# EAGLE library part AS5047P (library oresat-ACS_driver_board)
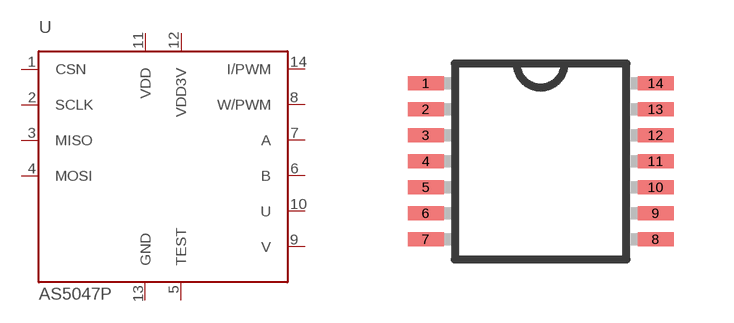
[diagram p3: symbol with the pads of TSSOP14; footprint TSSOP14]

Designator prefix U

## AS5047P  [TSSOP14]
1  CSN  in
2  SCLK  in
3  MISO  out
4  MOSI  in
5  TEST  pwr
6  B  out
7  A  out
8  W/PWM  out
9  V  out
10  U  out
11  VDD  pwr
12  VDD3V  pwr
13  GND  pwr
14  I/PWM  out

## Footprint TSSOP14 (pad centres in mm)
14-Lead Thin Shrink Small Outline Package [TSSOP] Source: Analog Devices .. 780914713ADD8704_0.pdf
smd 0.9 x 0.35: 1 -2.875,1.95; 2 -2.875,1.3; 3 -2.875,0.65; 4 -2.875,0; 5 -2.875,-0.65; 6 -2.875,-1.3; 7 -2.875,-1.95; 8 2.875,-1.95; 9 2.875,-1.3; 10 2.875,-0.65; 11 2.875,0; 12 2.875,0.65; 13 2.875,1.3; 14 2.875,1.95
